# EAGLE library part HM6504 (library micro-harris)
MICROCONTROLLER/MEMORY DEVICE
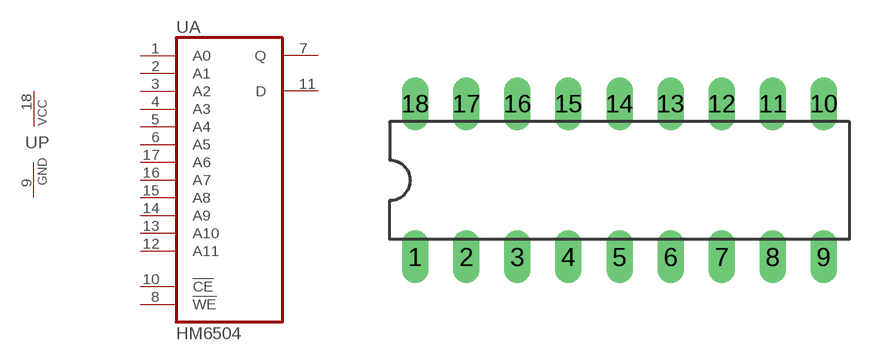
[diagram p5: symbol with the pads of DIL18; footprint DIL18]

Designator prefix U; gates A=HM6504 P=PWRN

## HM6504 (OC_FARNELL: unknown; OC_NEWARK: unknown)  [DIL18]
1  A:A0  in
2  A:A1  in
3  A:A2  in
4  A:A3  in
5  A:A4  in
6  A:A5  in
7  A:Q  hiz
8  A:!WE  in
9  P:GND  pwr
10  A:!CE  in
11  A:D  in
12  A:A11  in
13  A:A10  in
14  A:A9  in
15  A:A8  in
16  A:A7  in
17  A:A6  in
18  P:VCC  pwr

## Footprint DIL18 (pad centres in mm)
Dual In Line Package
drill 0.813 long: 1 -10.16,-3.81; 2 -7.62,-3.81; 3 -5.08,-3.81; 4 -2.54,-3.81; 5 0,-3.81; 6 2.54,-3.81; 7 5.08,-3.81; 8 7.62,-3.81; 9 10.16,-3.81; 10 10.16,3.81; 11 7.62,3.81; 12 5.08,3.81; 13 2.54,3.81; 14 0,3.81; 15 -2.54,3.81; 16 -5.08,3.81; 17 -7.62,3.81; 18 -10.16,3.81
